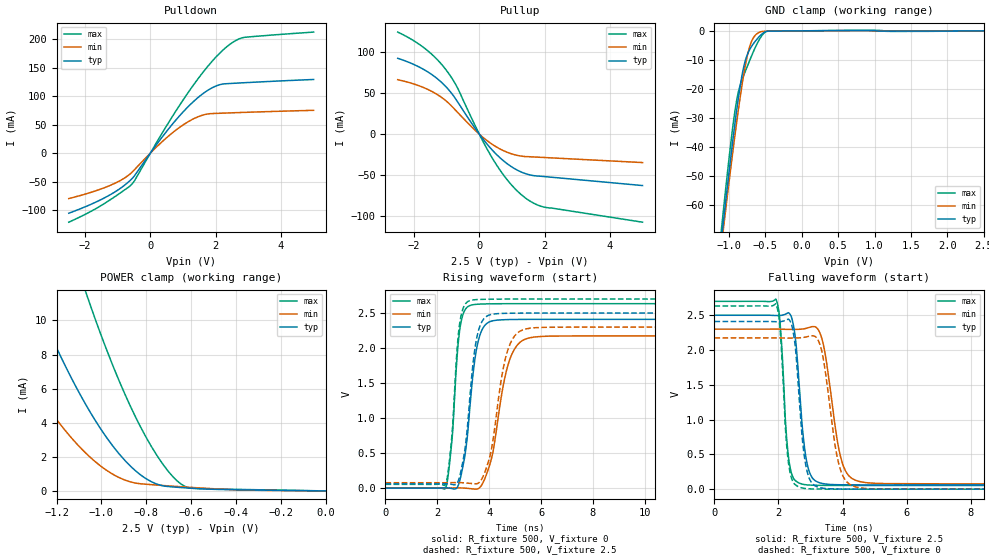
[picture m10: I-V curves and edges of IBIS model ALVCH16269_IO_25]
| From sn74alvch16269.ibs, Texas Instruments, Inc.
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[Model]   ALVCH16269_IO_25
Model_type  3-state
Enable   Active-Low
Vref =   0
Rref =   500
Cref =   30p
Vmeas =   1.25
| variable   typ   min   max
C_comp   7.68pF   6.80pF   8.82pF
| C_pullup   8.83pF   7.43pF   9.74pF
| C_pulldown   8.78pF   7.73pF   10.89pF
| C_tri-state   7.68pF   6.80pF   8.82pF
[Temperature Range]   40   100   -40
| Ambient temperature   25   85   -40
[Voltage range]   2.5   2.3   2.7
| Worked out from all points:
|   slope of the pulldown table from 0 to 0.375 V, typ, clamps not added: 12.8 ohm
|   slope of the pullup table from 0 to 0.375 V, typ, clamps not added: 20.3 ohm
|   GND clamp passes 1 mA (typ) near -0.54 V on its own axis
|   POWER clamp passes 1 mA (typ) near -0.83 V on its own axis
|   rising waveform, R_fixture 500, V_fixture 0: 20-80 % time 416ps typ, 615ps min, 294ps max; typ from 0 V to 2.41 V
|   falling waveform, R_fixture 500, V_fixture 2.5: 20-80 % time 265ps typ, 421ps min, 199ps max; typ from 2.5 V to 0.06 V
|   rising waveform, R_fixture 500, V_fixture 2.5: 20-80 % time 396ps typ, 562ps min, 285ps max; typ from 0.06 V to 2.5 V
|   falling waveform, R_fixture 500, V_fixture 0: 20-80 % time 256ps typ, 401ps min, 198ps max; typ from 2.41 V to 0 V
[GND Clamp]
| ALVCH16269_IO_25
|   Voltage   I(typ)   I(min)   I(max)
-2.5V     -419.2mA   -399.7mA   -437.1mA
-1.1V     -71.01mA   -73.15mA   -67.37mA
-1.08V    -66.47mA   -68.88mA   -62.56mA
-1.065V   -63.09mA   -65.7mA    -58.99mA
-920mV    -32.23mA   -36.3mA    -27.92mA
-875mV    -23.82mA   -27.91mA   -21.46mA
-820mV    -15.18mA   -18.51mA   -16.78mA
-770mV    -9.764mA   -11.23mA   -13.58mA
-710mV    -6.193mA   -4.989mA   -9.874mA
-590mV    -2.132mA   -586.8uA   -3.303mA
-475mV    -123.1uA   -125.6uA   -159.1uA
2.5V      60.98pA    21.96uA    -42.22uA
[POWER Clamp]
| ALVCH16269_IO_25
|   Voltage   I(typ)   I(min)   I(max)
-2.5V     64.19mA    43.37mA    95.45mA
-1.535V   19.59mA    11.55mA    33.75mA
-1.515V   18.83mA    11.03mA    32.66mA
-1.295V   11.23mA    5.98mA     21.43mA
-1.165V   7.441mA    3.605mA    15.55mA
-1.06V    4.844mA    2.097mA    11.29mA
-950mV    2.65mA     984.7uA    7.385mA
-845mV    1.148mA    453.2uA    4.26mA
-745mV    365.4uA    335.7uA    1.929mA
-655mV    206.9uA    253.8uA    504.1uA
-595mV    154.2uA    202.5uA    155.2uA
-31.15fV  60.98pA    310.2pA    10.68pA
[Pulldown]
| ALVCH16269_IO_25
|   Voltage   I(typ)   I(min)   I(max)
-2.5V     -105.6mA   -79.81mA   -121.4mA
-1.3V     -75.33mA   -58.3mA    -84.57mA
-860mV    -59.38mA   -46.13mA   -67.44mA
-560mV    -44.65mA   -33.4mA    -54.08mA
440mV     34.11mA    24.21mA    42.67mA
1.2V      84.08mA    56.61mA    110mA
1.545V    101.7mA    65.71mA    137.1mA
1.85V     113.5mA    69.42mA    158.7mA
2.125V    120.2mA    70.07mA    175.7mA
2.395V    122.2mA    70.66mA    189.5mA
2.88V     123.8mA    71.64mA    203.5mA
5V        129.4mA    75.25mA    212.7mA
[Pullup]
| ALVCH16269_IO_25
|   Voltage   I(typ)   I(min)   I(max)
-2.5V     92.66mA    66.56mA    124.7mA
-1.665V   78.11mA    56.19mA    104.5mA
-1.325V   68.92mA    49.28mA    92.52mA
-1.025V   58.04mA    40.84mA    78.82mA
-680mV    40.31mA    27.23mA    57.4mA
30mV      -1.639mA   -1.074mA   -2.414mA
440mV     -21.28mA   -13.54mA   -32.01mA
910mV     -37.73mA   -22.98mA   -58.46mA
1.38V     -47.71mA   -27.23mA   -76.95mA
1.69V     -50.76mA   -27.87mA   -84.79mA
2.005V    -51.81mA   -28.52mA   -89.22mA
5V        -62.74mA   -34.67mA   -107.5mA
[Ramp]
| ALVCH16269_IO_25
| variable   typ   min   max
dV/dt_r   1.45/4.23E-10   1.31/6.25E-10   1.59/3.00E-10
dV/dt_f   1.49/2.71E-10   1.36/4.35E-10   1.61/2.09E-10
R_load = 500
[Rising Waveform]
| ALVCH16269_IO_25
R_fixture =   500
C_fixture =   0
L_fixture =   0
V_fixture =   0
V_fixture_min = 0
V_fixture_max = 0
|   Time   V(typ)   V(min)   V(max)
0s        82.22pV    2.599nV    65.98pV
2.32ns    3.125mV    -439.4uV   5.504mV
2.57ns    -7.471mV   1.597mV    708.5mV
2.875ns   120mV      2.284mV    2.287V
3.135ns   658.9mV    -3.083mV   2.579V
3.42ns    1.759V     -13.62mV   2.622V
4.04ns    2.379V     353.6mV    2.632V
4.84ns    2.408V     1.88V      2.634V
5.74ns    2.41V      2.158V     2.634V
50ns      2.41V      2.175V     2.634V
[Falling Waveform]
| ALVCH16269_IO_25
R_fixture =   500
C_fixture =   0
L_fixture =   0
V_fixture =   2.5
V_fixture_min = 2.3
V_fixture_max = 2.7
|   Time   V(typ)   V(min)   V(max)
0s        2.5V       2.3V       2.7V
1.925ns   2.496V     2.3V       2.724V
2.055ns   2.497V     2.3V       2.358V
2.335ns   2.529V     2.297V     384.6mV
2.535ns   2.141V     2.297V     120.5mV
2.865ns   435.4mV    2.312V     62.9mV
3.36ns    82.79mV    2.157V     54.83mV
4.03ns    62.71mV    328.1mV    53.44mV
4.77ns    60.84mV    91.63mV    53.23mV
50ns      60.4mV     76.46mV    53.19mV
[Rising Waveform]
| ALVCH16269_IO_25
R_fixture =   500
C_fixture =   0
L_fixture =   0
V_fixture =   2.5
V_fixture_min = 2.3
V_fixture_max = 2.7
|   Time   V(typ)   V(min)   V(max)
0s        60.4mV     76.46mV    53.19mV
2.32ns    63.18mV    76.12mV    58.74mV
2.565ns   52.4mV     78.09mV    760.2mV
2.865ns   170.8mV    77.8mV     2.358V
3.37ns    1.758V     64.01mV    2.687V
3.625ns   2.294V     83.24mV    2.695V
4.025ns   2.475V     448.8mV    2.698V
4.76ns    2.497V     2.015V     2.7V
5.58ns    2.5V       2.284V     2.7V
50ns      2.5V       2.3V       2.7V
[Falling Waveform]
| ALVCH16269_IO_25
R_fixture =   500
C_fixture =   0
L_fixture =   0
V_fixture =   0
V_fixture_min = 0
V_fixture_max = 0
|   Time   V(typ)   V(min)   V(max)
0s        2.41V      2.175V     2.634V
1.92ns    2.407V     2.175V     2.661V
2.045ns   2.408V     2.174V     2.322V
2.33ns    2.437V     2.172V     318.7mV
2.52ns    2.065V     2.173V     66.17mV
2.83ns    403.7mV    2.185V     9.875mV
3.34ns    17.54mV    2.009V     1.392mV
3.975ns   1.751mV    228.1mV    222.4uV
4.665ns   326.8uV    12.16mV    38.27uV
50ns      425.4nV    696nV      263nV
